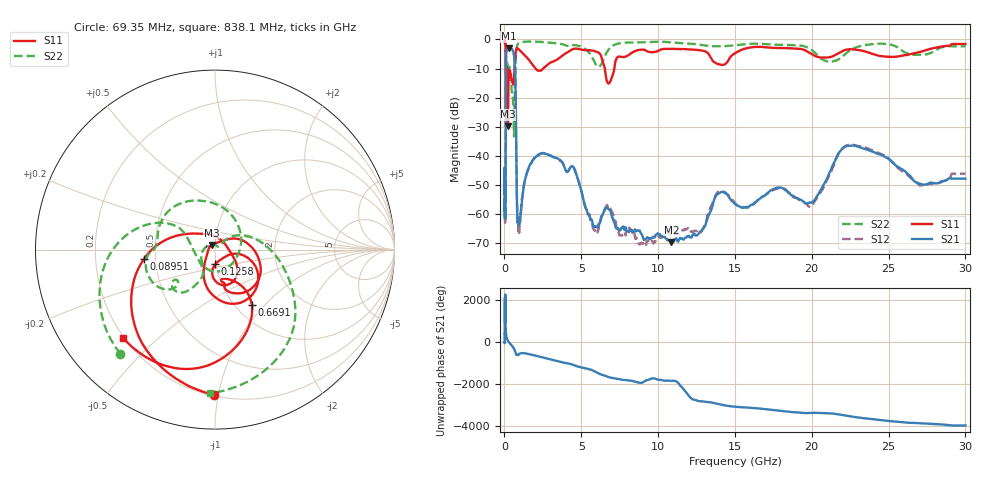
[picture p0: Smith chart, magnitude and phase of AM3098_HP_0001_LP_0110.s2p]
! Date/Time: Thu, Feb 28, 2019 8:31 AM
! Network Analyzer: Agilent Technologies E8364B Rev: A.07.50.67
! Sweep from 0.010 to 30.000 GHz, 1601 Points, Sweep Type: LOG
! Power Supply: 5.023 V, 0.002 A
# Hz S DB R 50
!freq MagS11 AngS11 MagS21 AngS21 MagS12 AngS12 MagS22 AngS22
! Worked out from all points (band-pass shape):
!   1601 points, 10 MHz to 30 GHz, reference 50 ohm
!   highest |S21| = -3.09 dB at 266.5 MHz (marker M1); lowest = -69.7 dB at 10.86 GHz (marker M2)
!   |S21| within 3 dB of the highest: 104.5 MHz to 640.7 MHz (536.1 MHz wide, 144 % of centre)
!   lowest |S11| = -30.0 dB at 227 MHz (marker M3), VSWR 1.07, Z = 48.1 + j2.45 ohm
!   |S11| at or under -10 dB: 175.9 MHz to 655.5 MHz (479.6 MHz wide, 115 % of centre); 2.028 GHz to 2.521 GHz (493.7 MHz wide, 21.7 % of centre); 6.529 GHz to 7.149 GHz (620.2 MHz wide, 9.07 % of centre)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
!   |S22| runs from -33.4 to -0.6 dB; largest |S21 - S12| = 0.0094
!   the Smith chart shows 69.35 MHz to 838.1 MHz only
!   S11 on the Smith chart (normalised r, x): 69.35 MHz: 0.21, -0.97; 89.51 MHz: 0.43, -0.05; 125.8 MHz: 0.99, -0.16; 669.1 MHz: 1.19, -0.84; 838.1 MHz: 0.20, -0.39
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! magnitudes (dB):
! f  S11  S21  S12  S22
! 10 MHz  -0.3  -48.7  -46.0  -0.6
! 38.04 MHz  -0.5  -59.6  -62.1  -0.9
! 69.35 MHz  -1.8  -55.9  -53.1  -2.1
! 89.51 MHz  -8.0  -18.9  -18.8  -9.5
! 98.93 MHz  -24.0  -7.8  -7.8  -16.9
! 125.8 MHz  -21.8  -4.2  -4.2  -10.8
! 144.7 MHz  -13.3  -3.6  -3.6  -10.1
! 185.8 MHz  -11.3  -3.5  -3.5  -8.1
! 227 MHz  -30.0  -3.2  -3.1  -9.5
! 266.5 MHz  -14.4  -3.1  -3.1  -9.7
! 550.5 MHz  -15.5  -3.9  -3.9  -20.4
! 620.7 MHz  -13.1  -5.3  -5.2  -33.3
! 669.1 MHz  -8.7  -8.0  -8.0  -20.8
! 838.1 MHz  -3.0  -60.7  -60.3  -1.9
! 2.084 GHz  -10.4  -40.2  -40.2  -0.8
! 4.458 GHz  -3.3  -43.8  -43.6  -1.9
! 5.87 GHz  -4.0  -64.4  -65.7  -7.8
! 7.926 GHz  -5.8  -65.3  -66.1  -1.1
! 10.86 GHz  -3.2  -69.7  -67.0  -1.0
! 19.9 GHz  -4.8  -56.1  -57.7  -3.2
! 22.67 GHz  -3.4  -36.5  -36.3  -3.2
! 30 GHz  -1.6  -48.0  -46.2  -2.3
